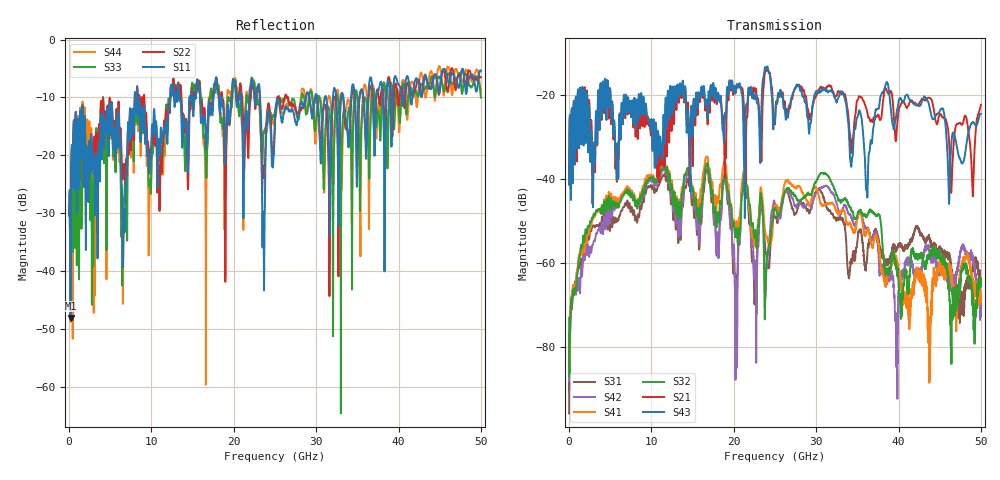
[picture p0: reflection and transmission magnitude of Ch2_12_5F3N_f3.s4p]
!Agilent Technologies,N5247A,US51170199,A.09.90.13
!Agilent N5247A: A.09.90.13
!Date: Tuesday, December 08, 2015 12:23:33
!Correction: S11(Full 4 Port(1,2,3,4))
!S12(Full 4 Port(1,2,3,4))
!S13(Full 4 Port(1,2,3,4))
!S14(Full 4 Port(1,2,3,4))
!S21(Full 4 Port(1,2,3,4))
!S22(Full 4 Port(1,2,3,4))
!S23(Full 4 Port(1,2,3,4))
!S24(Full 4 Port(1,2,3,4))
!S31(Full 4 Port(1,2,3,4))
!S32(Full 4 Port(1,2,3,4))
!S33(Full 4 Port(1,2,3,4))
!S34(Full 4 Port(1,2,3,4))
!S41(Full 4 Port(1,2,3,4))
!S42(Full 4 Port(1,2,3,4))
!S43(Full 4 Port(1,2,3,4))
!S44(Full 4 Port(1,2,3,4))
!S4P File: Measurements: <S11,S12,S13,S14>,
!<S21,S22,S23,S24>,
!<S31,S32,S33,S34>,
!<S41,S42,S43,S44>:
# Hz S  dB  R 50
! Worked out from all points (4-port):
!   3201 points, 10 MHz to 50 GHz, reference 50 ohm
!   strongest paths, dB at 10 MHz, 12.51 GHz, 25 GHz, 37.5 GHz, 50 GHz:
!     S43: -41.4, -20.3, -26.1, -23.4, -24.5
!     S21: -41.3, -21.6, -26.9, -24.7, -22.4
!     S32: -73.0, -41.5, -47.2, -48.4, -63.7
!     S41: -78.5, -40.9, -46.2, -54.5, -68.8
!     S42: -78.4, -41.6, -45.9, -56.1, -72.0
!     S31: -95.8, -43.3, -49.1, -54.0, -64.2
!   lowest |S11| = -48.1 dB at 181.8 MHz (marker M1), VSWR 1.01, Z = 50.1 - j0.384 ohm
!   |S11| at or under -10 dB: start of sweep to 7.973 GHz; 8.34 GHz to 12.28 GHz (3.945 GHz wide, 38.3 % of centre); 23.19 GHz to 28.79 GHz (5.6 GHz wide, 21.5 % of centre)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
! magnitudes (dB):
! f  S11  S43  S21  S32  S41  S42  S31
! 10 MHz  -30.2  -41.4  -41.3  -73.0  -78.5  -78.4  -95.8
! 181.8 MHz  -48.1  -30.8  -30.6  -71.7  -70.7  -72.8  -73.4
! 16.68 GHz  -17.9  -21.1  -21.8  -36.6  -34.8  -36.9  -38.2
! 20.29 GHz  -10.3  -18.8  -18.4  -52.6  -50.5  -65.4  -63.6
! 21.3 GHz  -14.8  -38.7  -24.8  -38.8  -37.7  -39.1  -39.5
! 31.18 GHz  -9.9  -19.1  -18.6  -38.9  -46.0  -41.7  -46.3
! 50 GHz  -5.4  -24.5  -22.4  -63.7  -68.8  -72.0  -64.2
